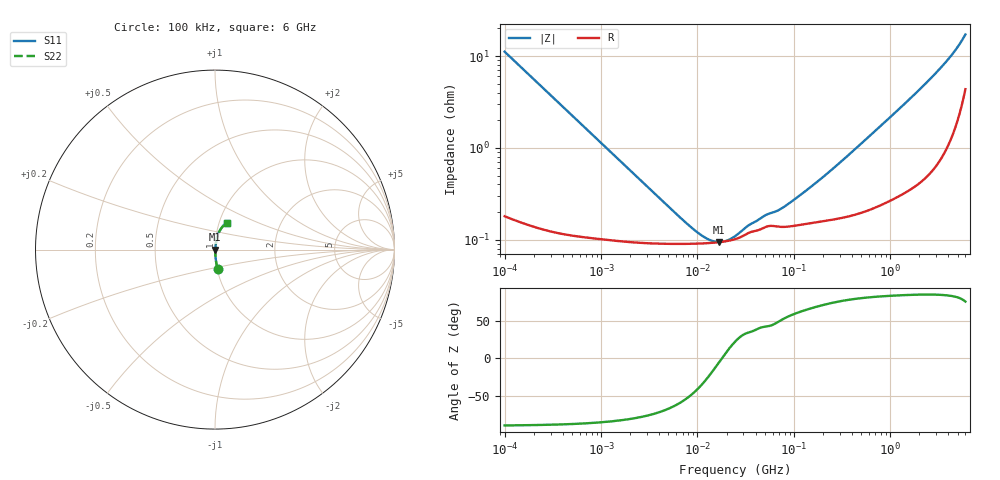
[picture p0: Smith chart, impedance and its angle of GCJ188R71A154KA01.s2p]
!Murata Part Number: GCJ188R71A154KA01
!These Parameters are Measured in Series Mode Connection
!Data Generated on Mar 13, 2026
!  o--ll--o
!Port1  Port2
!  o------o
!Operation Temp=25[degC], DC Bias Voltage=0[V]
!Freq. Start=100[kHz] Stop=6[GHz] 401[Steps]
# Hz S RI R 50
!Freq.(Hz) S11(Real) S11(Imag) S21(Real) S21(Imag) S12(Real) S12(Imag) S22(Real) S22(Imag)
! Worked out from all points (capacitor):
!   401 points, 100 kHz to 6 GHz, reference 50 ohm
!   read as one part in series: C = 142 nF near 105.7 kHz
!   lowest |Z| = 94.4 mohm at 16.67 MHz (marker M1)
!   series resonance near 17.89 MHz, so ESL is about 560 pH
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100000  0.014 -0.1098  0.986 0.1098  0.986 0.1098  0.014 -0.1098
105655  0.0127 -0.1041  0.9873 0.1041  0.9873 0.1041  0.0127 -0.1041
228224  0.00372 -0.0489  0.9963 0.0489  0.9963 0.0489  0.00372 -0.0489
631452  0.00139 -0.0178  0.9986 0.0178  0.9986 0.0178  0.00139 -0.0178
3987316  0.000912 -0.00272  0.9991 0.00272  0.9991 0.00272  0.000912 -0.00272
7302625  0.000901 -0.0013  0.9991 0.0013  0.9991 0.0013  0.000901 -0.0013
1.015836e7  0.000907 -0.000762  0.9991 0.000762  0.9991 0.000762  0.000907 -0.000762
1.337449e7  0.00092 -0.000376  0.9991 0.000376  0.9991 0.000376  0.00092 -0.000376
1.666634e7  0.000938 -9.02e-05  0.9991 9.02e-05  0.9991 9.02e-05  0.000938 -9.02e-05
2.020496e7  0.000966 0.000156  0.999 -0.000156  0.999 -0.000156  0.000966 0.000156
2.517799e7  0.00102 0.000445  0.999 -0.000445  0.999 -0.000445  0.00102 0.000445
3.314933e7  0.00117 0.000785  0.9988 -0.000785  0.9988 -0.000785  0.00117 0.000785
4.872031e7  0.00135 0.0012  0.9987 -0.0012  0.9987 -0.0012  0.00135 0.0012
6.593397e7  0.00139 0.00149  0.9986 -0.00149  0.9986 -0.00149  0.00139 0.00149
7.776452e7  0.00138 0.00178  0.9986 -0.00178  0.9986 -0.00178  0.00138 0.00178
1.546735e8  0.00153 0.00354  0.9985 -0.00354  0.9985 -0.00354  0.00153 0.00354
3.076454e8  0.00176 0.00684  0.9982 -0.00684  0.9982 -0.00684  0.00176 0.00684
9.76689e8  0.00306 0.0209  0.9969 -0.0209  0.9969 -0.0209  0.00306 0.0209
1.889928e9  0.00553 0.04  0.9945 -0.04  0.9945 -0.04  0.00553 0.04
3.100717e9  0.0112 0.0671  0.9888 -0.0671  0.9888 -0.0671  0.0112 0.0671
4.557193e9  0.0261 0.1048  0.9739 -0.1048  0.9739 -0.1048  0.0261 0.1048
6e9  0.0655 0.1488  0.9345 -0.1488  0.9345 -0.1488  0.0655 0.1488
